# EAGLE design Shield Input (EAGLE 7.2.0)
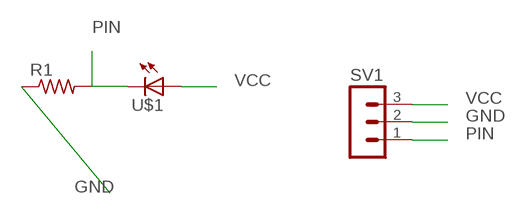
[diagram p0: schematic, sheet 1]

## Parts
R1  RESISTOR1206  [1206]
SV1  MA03-1  [MA03-1]
U$1  LED5MM  [5MM]

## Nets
GND: R1.1 SV1.2
PIN: R1.2 SV1.1 U$1.OUT(C)
VCC: SV1.3 U$1.IN(A)

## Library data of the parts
R1 = 01_FAB_Hello:RESISTOR
SV1 = con-lstb:MA03-1: PIN HEADER; OC_FARNELL: unknown; OC_NEWARK: unknown
U$1 = 01_FAB_Hello:LED

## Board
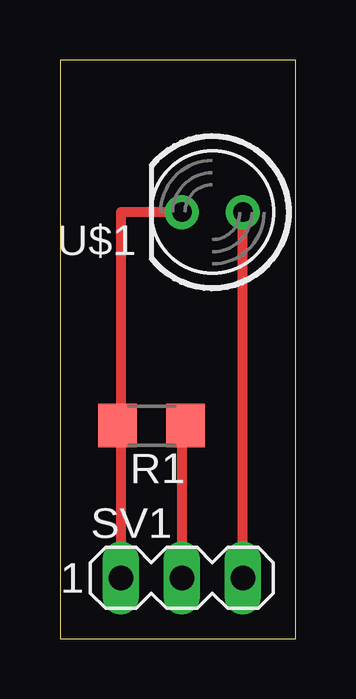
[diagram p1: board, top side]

Size 9.83 x 24.12 mm. Coordinates in mm from the lower left corner, seen from the top.
Outline: 0,0 9.83,0 9.83,24.12 0,24.12 0,0
Copper layers (1*16): Top 0.035mm / dielectric 1.5mm / Bottom 0.035mm
Design rules "default": minimum track width 10mil, minimum drill 24mil, track to track 8mil, track to pad 8mil, pad to pad 8mil, via to via 8mil, smd to smd 8mil, copper to edge 40mil, drill to drill 8mil, minimum pad ring 10mil, minimum via ring 8mil, stop-mask expansion 4mil, vias tented up to drill 0mil, thermal gap 10mil

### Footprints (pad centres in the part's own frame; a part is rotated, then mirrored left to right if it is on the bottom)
1206 = smd 1.6 x 1.803: 1 -1.422,0; 2 1.422,0
MA03-1 = drill 1.016 long: 1 -2.54,0; 2 0,0; 3 2.54,0
5MM = drill 0.813 pad 1.422: IN -1.27,0; OUT 1.27,0

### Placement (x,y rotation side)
R1  3.81,8.89 180 top
SV1  5.08,2.54 0 top
U$1  6.35,17.78 180 top

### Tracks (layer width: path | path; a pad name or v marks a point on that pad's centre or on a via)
GND
  Top 0.406: R1.1 5.08,8.89 SV1.2
PIN
  Top 0.406: U$1.OUT 2.54,17.78 2.54,8.89 | R1.2 2.54,8.89 | 2.54,8.89 SV1.1
VCC
  Top 0.406: SV1.3 U$1.IN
